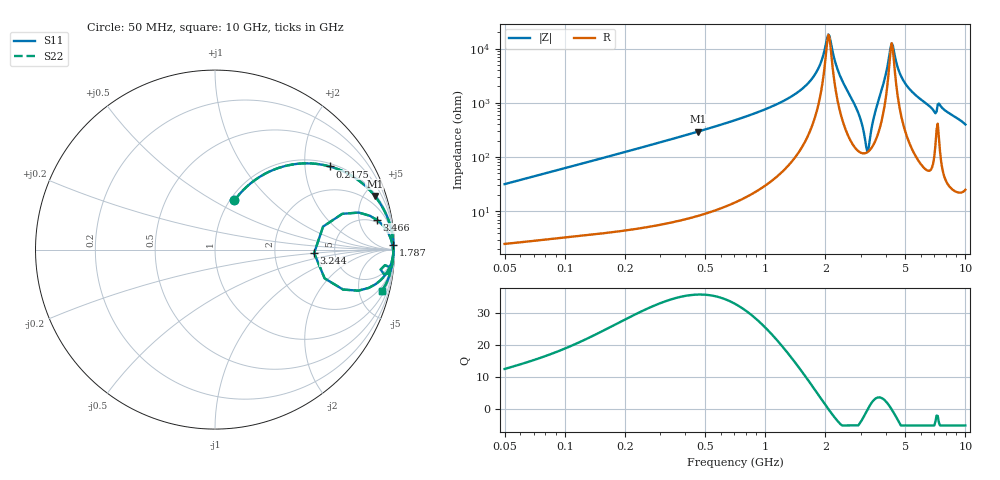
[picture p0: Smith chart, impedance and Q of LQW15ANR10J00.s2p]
!Murata Part Number: LQW15ANR10J00
!These Parameters are Measured in Series Mode Connection
!  o--[Z]--o
!Port1  Port2
!  o-------o
!Freq. Start=50[MHz] Stop=10[GHz], 401[Steps]
# Hz S RI R 50
!Freq.(Hz)	S 11(Real)	S 11(Imag)	S 21(Real)	S 21(Imag)	S 12(Real)	S 12(Imag)	S 22(Real)	S 22(Imag)
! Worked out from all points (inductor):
!   401 points, 50 MHz to 10 GHz, reference 50 ohm
!   read as one part in series: L = 99.7 nH near 51.34 MHz
!   highest Q = 35.8 at 462.8 MHz (marker M1), where L = 101 nH
!   self-resonance near 2.067 GHz
!   S11 on the Smith chart (normalised r, x): 50 MHz: 1.05, +0.63; 217.5 MHz: 1.09, +2.70; 1.787 GHz: 13, +69; 3.244 GHz: 3.46, -0.19; 3.466 GHz: 4, +9; 10 GHz: 1.50, -7.94
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5e7  0.1085 0.274  0.8915 -0.274  0.8915 -0.274  0.1085 0.274
1.214486e8  0.3685 0.4595  0.6315 -0.4595  0.6315 -0.4595  0.3685 0.4595
2.175233e8  0.6406 0.463  0.3594 -0.463  0.3594 -0.463  0.6406 0.463
2.949953e8  0.7648 0.4093  0.2352 -0.4093  0.2352 -0.4093  0.7648 0.4093
4.628099e8  0.8901 0.2991  0.1099 -0.2991  0.1099 -0.2991  0.8901 0.2991
7.071068e8  0.9524 0.1983  0.0476 -0.1983  0.0476 -0.1983  0.9524 0.1983
1.26648e9  0.9877 0.0863  0.0123 -0.0863  0.0123 -0.0863  0.9877 0.0863
1.717543e9  0.994 0.0349  0.00601 -0.0349  0.00601 -0.0349  0.994 0.0349
1.787167e9  0.9944 0.028  0.00565 -0.028  0.00565 -0.028  0.9944 0.028
2.040286e9  0.9947 0.00345  0.00535 -0.00345  0.00535 -0.00345  0.9947 0.00345
2.095058e9  0.9945 -0.00192  0.0055 0.00192  0.0055 0.00192  0.9945 -0.00192
2.329253e9  0.9927 -0.0264  0.00734 0.0264  0.00734 0.0264  0.9927 -0.0264
2.917498e9  0.9503 -0.1389  0.0497 0.1389  0.0497 0.1389  0.9503 -0.1389
3.117263e9  0.7991 -0.2288  0.2009 0.2288  0.2009 0.2288  0.7991 -0.2288
3.243629e9  0.5524 -0.0195  0.4476 0.0195  0.4476 0.0195  0.5524 -0.0195
3.465724e9  0.9032 0.1646  0.0968 -0.1646  0.0968 -0.1646  0.9032 0.1646
4.171863e9  0.9911 0.00969  0.00888 -0.00969  0.00888 -0.00969  0.9911 0.00969
4.34098e9  0.9924 -0.00425  0.00759 0.00425  0.00759 0.00425  0.9924 -0.00425
4.826234e9  0.9928 -0.0341  0.00717 0.0341  0.00717 0.0341  0.9928 -0.0341
5.657692e9  0.9894 -0.0716  0.0106 0.0716  0.0106 0.0716  0.9894 -0.0716
6.901252e9  0.9691 -0.129  0.0309 0.129  0.0309 0.129  0.9691 -0.129
1e10  0.928 -0.2291  0.072 0.2291  0.072 0.2291  0.928 -0.2291
